(* Logix 5000 AddOnInstructionDefinition export SPEL_Init; software revision 30.01 *)

ADD_ON_INSTRUCTION SPEL_ExecCmd   (* revision 1.2 *)
// Executes a command in the robot controller.  Normally this is called by higher level AOIs.
VAR_INPUT
   Start : BOOL; {required}
   MaxTime : DINT := 3000; {required}
END_VAR
VAR_OUTPUT
   InCycle : BOOL; {access Read Only, visible}
   Done : BOOL; {access Read Only, visible}
   Error : BOOL; {access Read Only, visible}
END_VAR
VAR_IN_OUT
   ExtInputs : AB:ETHERNET_MODULE_INT_128Bytes:I:0; {required}
        .DATA[0].0   // ExtCmdGet
        .DATA[0].1   // ExtRespSet
        .DATA[0].2   // ExtCmdResult
        .DATA[0].3   // ExtError
   ExtOutputs : AB:ETHERNET_MODULE_INT_128Bytes:O:0; {required}
        .DATA[0].0   // ExtCmdSet
        .DATA[0].1   // ExtRespGet
        .DATA[0].2   // ExtCmdReset
END_VAR
VAR_INPUT
   Cmd : INT; {required}
   CmdParam1 : INT; {required}
   CmdParam2 : INT; {required}
   CmdParam3 : INT; {required}
   CmdParam4 : INT; {required}
   CmdParam5 : INT; {required}
   CmdParam6 : INT; {required}
   CmdParam7 : INT; {required}
END_VAR
VAR_OUTPUT
   CmdEcho : INT; {access Read Only, visible}
   Resp1 : INT; {access Read Only, visible}
   Resp2 : INT; {access Read Only, visible}
   Resp3 : INT; {access Read Only, visible}
   Resp4 : INT; {access Read Only, visible}
   Resp5 : INT; {access Read Only, visible}
   Resp6 : INT; {access Read Only, visible}
   Resp7 : INT; {access Read Only, visible}
   ErrCode1 : INT; {access Read Only, visible}
   ErrCode2 : INT; {access Read Only, visible}
END_VAR
VAR
   ExtReset : BOOL; {access None}
   ExtError : BOOL; {access None}
   ExtCmdSet : BOOL; {access None}   // Cmd Ready
   ExtCmdGet : BOOL; {access None}   // Cmd Received
   CmdXferDone : BOOL; {access None}
   ExtRespSet : BOOL; {access None}   // Resp Ready
   RespXferDone : BOOL; {access None}
   ExtCmdResult : BOOL; {access None}   // Normal or Error?
   TmrCmdDataRdy : TIMER := (PRE := 5); {access None}
   OneShotDoneOff : BOOL; {access None}
   OneShotStart : BOOL; {access None}
   StartInit : BOOL; {access None}
   OneShotStartError : BOOL; {access None}
   TmrCycle : TIMER := (PRE := 5000); {access None}
   OneshotTmrPreset : BOOL; {access None}
   TmrCmdSet : TIMER := (PRE := 20); {access None}
   OnShotCmdDataXfer : BOOL; {access None}
   OneShotRespDataXfer : BOOL; {access None}
   OneShotDataRdy : BOOL; {access None}
   OtherCmdInCycle : BOOL; {access None}
   s : BOOL; {access None}
   OneShotUnsetCmdIncycle : BOOL; {access None}
   OneShotSetCmdIncycle : BOOL; {access None}
   OneShotSetOtherCmdInCycleError : BOOL; {access None}
   OneShotSetBit : BOOL; {access None}
   MaxTimeError : BOOL; {access None}
END_VAR

ROUTINE Logic   (* ladder *)
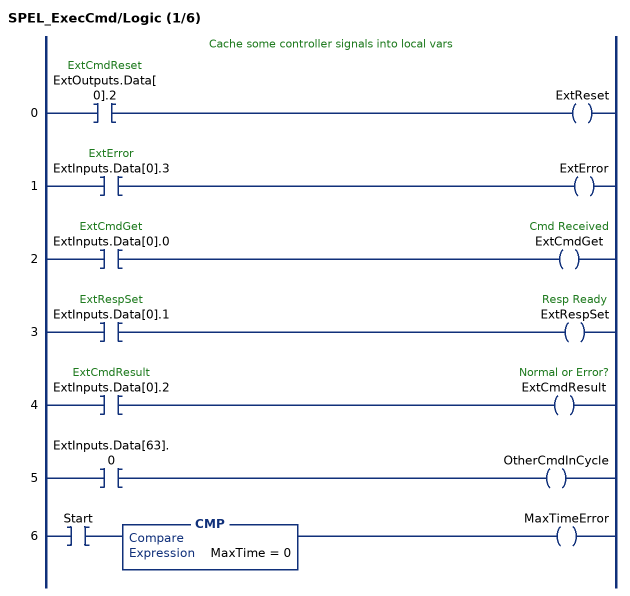
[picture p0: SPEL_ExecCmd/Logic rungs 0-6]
   // Cache some controller signals into local vars
   0: XIC(ExtOutputs.Data[0].2)OTE(ExtReset);
   1: XIC(ExtInputs.Data[0].3)OTE(ExtError);
   2: XIC(ExtInputs.Data[0].0)OTE(ExtCmdGet);
   3: XIC(ExtInputs.Data[0].1)OTE(ExtRespSet);
   4: XIC(ExtInputs.Data[0].2)OTE(ExtCmdResult);
   5: XIC(ExtInputs.Data[63].0)OTE(OtherCmdInCycle);
   6: XIC(Start)CMP(MaxTime = 0)OTE(MaxTimeError);
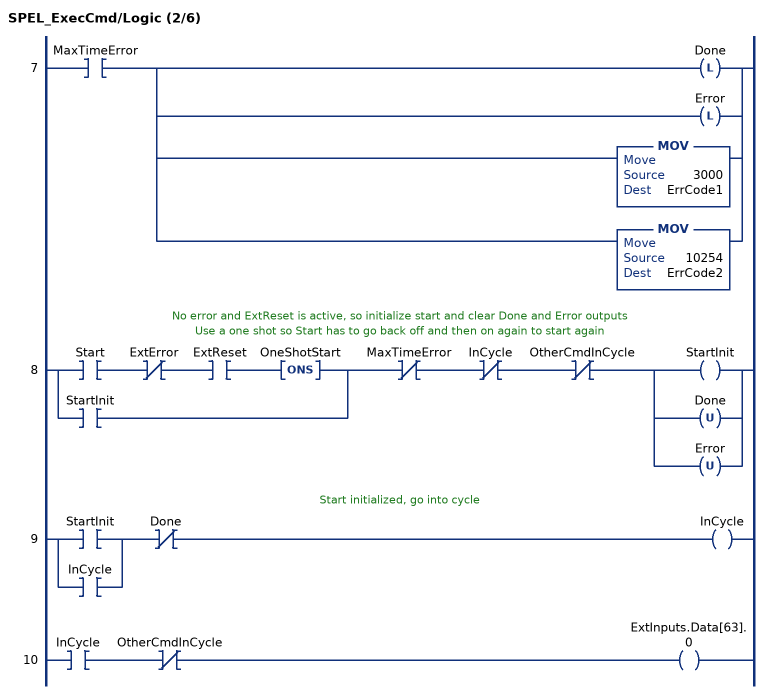
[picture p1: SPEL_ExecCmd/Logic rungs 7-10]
   7: XIC(MaxTimeError)[OTL(Done) ,OTL(Error) ,MOV(3000,ErrCode1) ,MOV(10254,ErrCode2) ];
   // No error and ExtReset is active, so initialize start and clear Done and Error outputs
   // Use a one shot so Start has to go back off and then on again to start again
   8: [XIC(Start) XIO(ExtError) XIC(ExtReset) ONS(OneShotStart) ,XIC(StartInit) ]XIO(MaxTimeError)XIO(InCycle)XIO(OtherCmdInCycle)[OTE(StartInit) ,OTU(Done) ,OTU(Error) ];
   // Start initialized, go into cycle
   9: [XIC(StartInit) ,XIC(InCycle) ]XIO(Done)OTE(InCycle);
   10: XIC(InCycle)XIO(OtherCmdInCycle)OTE(ExtInputs.Data[63].0);
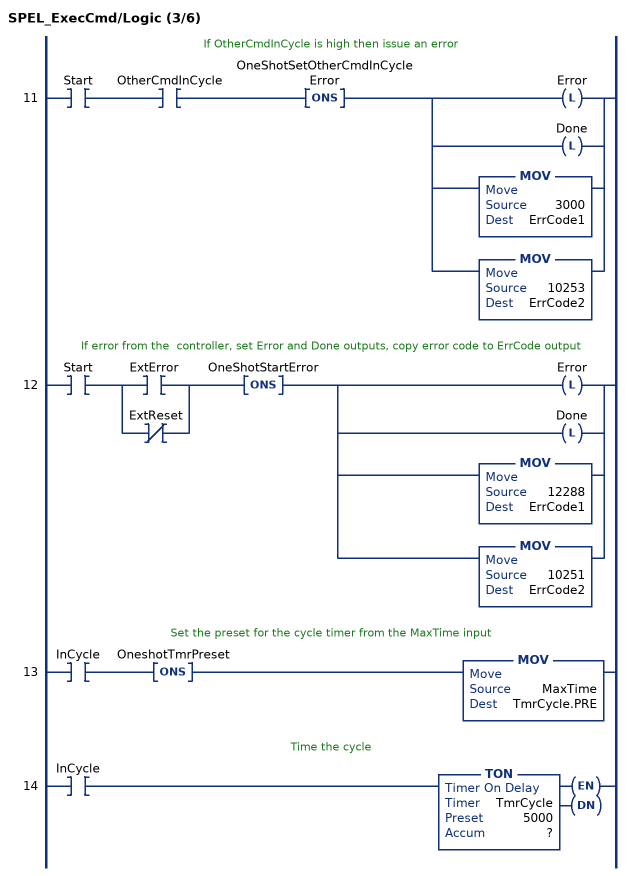
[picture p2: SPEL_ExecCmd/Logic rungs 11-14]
   // If OtherCmdInCycle is high then issue an error
   11: XIC(Start)XIC(OtherCmdInCycle)ONS(OneShotSetOtherCmdInCycleError)[OTL(Error) ,OTL(Done) ,MOV(3000,ErrCode1) ,MOV(10253,ErrCode2) ];
   // If error from the  controller, set Error and Done outputs, copy error code to ErrCode output
   12: XIC(Start)[XIC(ExtError) ,XIO(ExtReset) ]ONS(OneShotStartError)[OTL(Error) ,OTL(Done) ,MOV(12288,ErrCode1) ,MOV(10251,ErrCode2) ];
   // Set the preset for the cycle timer from the MaxTime input
   13: XIC(InCycle)ONS(OneshotTmrPreset)MOV(MaxTime,TmrCycle.PRE);
   // Time the cycle
   14: XIC(InCycle)TON(TmrCycle,?,?);
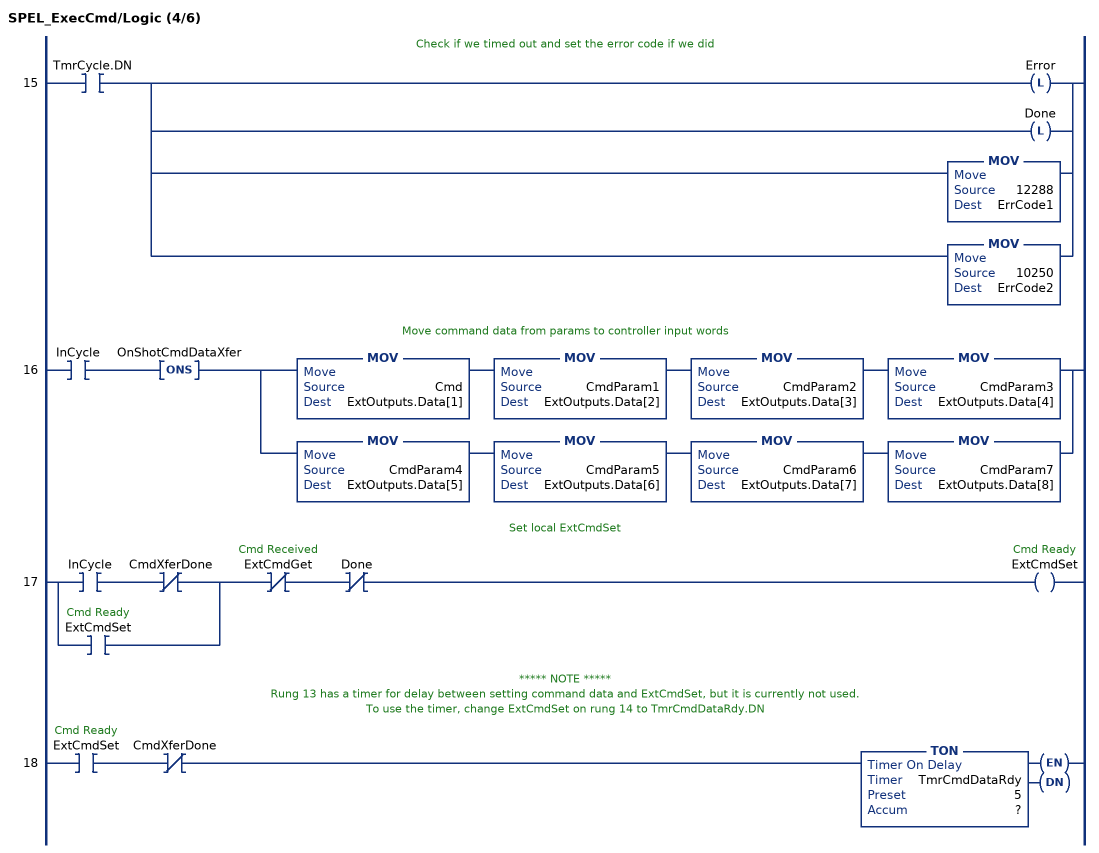
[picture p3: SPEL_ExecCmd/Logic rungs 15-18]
   // Check if we timed out and set the error code if we did
   15: XIC(TmrCycle.DN)[OTL(Error) ,OTL(Done) ,MOV(12288,ErrCode1) ,MOV(10250,ErrCode2) ];
   // Move command data from params to controller input words
   16: XIC(InCycle)ONS(OnShotCmdDataXfer)[MOV(Cmd,ExtOutputs.Data[1]) MOV(CmdParam1,ExtOutputs.Data[2]) MOV(CmdParam2,ExtOutputs.Data[3]) MOV(CmdParam3,ExtOutputs.Data[4]) ,MOV(CmdParam4,ExtOutputs.Data[5]) MOV(CmdParam5,ExtOutputs.Data[6]) MOV(CmdParam6,ExtOutputs.Data[7]) MOV(CmdParam7,ExtOutputs.Data[8]) ];
   // Set local ExtCmdSet
   17: [XIC(InCycle) XIO(CmdXferDone) ,XIC(ExtCmdSet) ]XIO(ExtCmdGet)XIO(Done)OTE(ExtCmdSet);
   // ***** NOTE *****
   // Rung 13 has a timer for delay between setting command data and ExtCmdSet, but it is currently not used.
   // To use the timer, change ExtCmdSet on rung 14 to TmrCmdDataRdy.DN
   18: XIC(ExtCmdSet)XIO(CmdXferDone)TON(TmrCmdDataRdy,?,?);
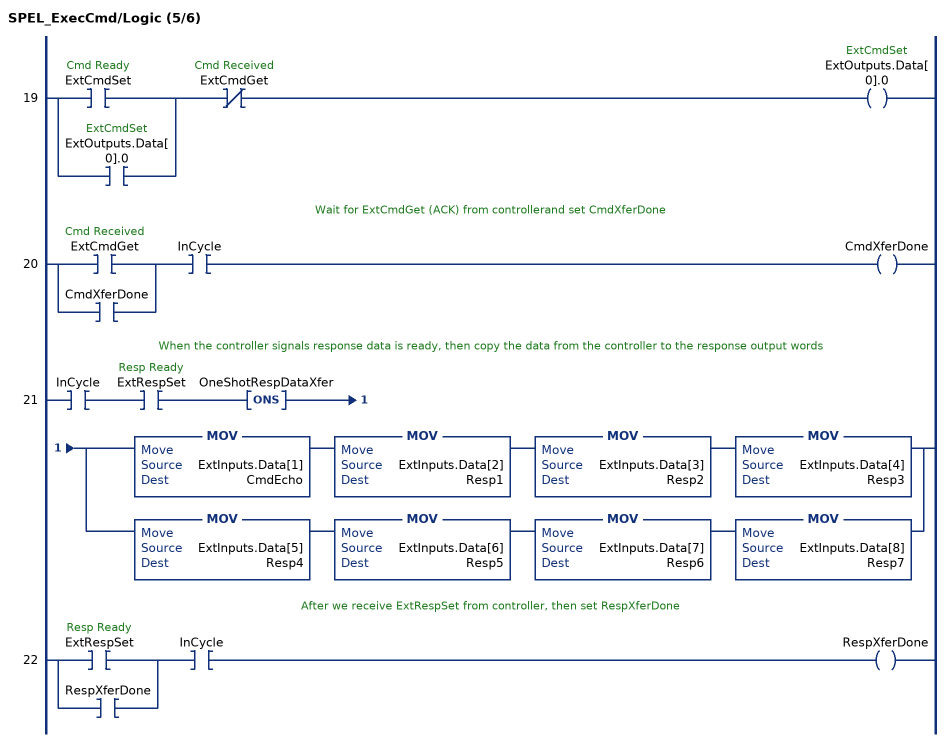
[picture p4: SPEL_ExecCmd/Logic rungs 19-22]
   19: [XIC(ExtCmdSet) ,XIC(ExtOutputs.Data[0].0) ]XIO(ExtCmdGet)OTE(ExtOutputs.Data[0].0);
   // Wait for ExtCmdGet (ACK) from controllerand set CmdXferDone
   20: [XIC(ExtCmdGet) ,XIC(CmdXferDone) ]XIC(InCycle)OTE(CmdXferDone);
   // When the controller signals response data is ready, then copy the data from the controller to the response output words
   21: XIC(InCycle)XIC(ExtRespSet)ONS(OneShotRespDataXfer)[MOV(ExtInputs.Data[1],CmdEcho) MOV(ExtInputs.Data[2],Resp1) MOV(ExtInputs.Data[3],Resp2) MOV(ExtInputs.Data[4],Resp3) ,MOV(ExtInputs.Data[5],Resp4) MOV(ExtInputs.Data[6],Resp5) MOV(ExtInputs.Data[7],Resp6) MOV(ExtInputs.Data[8],Resp7) ];
   // After we receive ExtRespSet from controller, then set RespXferDone
   22: [XIC(ExtRespSet) ,XIC(RespXferDone) ]XIC(InCycle)OTE(RespXferDone);
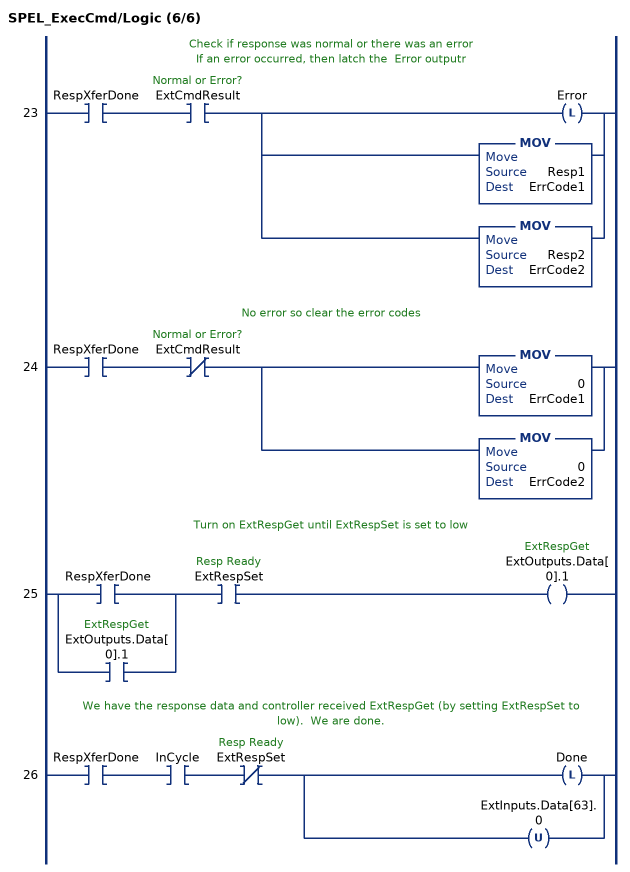
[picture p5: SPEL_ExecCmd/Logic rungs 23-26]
   // Check if response was normal or there was an error
   // If an error occurred, then latch the  Error outputr
   23: XIC(RespXferDone)XIC(ExtCmdResult)[OTL(Error) ,MOV(Resp1,ErrCode1) ,MOV(Resp2,ErrCode2) ];
   // No error so clear the error codes
   24: XIC(RespXferDone)XIO(ExtCmdResult)[MOV(0,ErrCode1) ,MOV(0,ErrCode2) ];
   // Turn on ExtRespGet until ExtRespSet is set to low
   25: [XIC(RespXferDone) ,XIC(ExtOutputs.Data[0].1) ]XIC(ExtRespSet)OTE(ExtOutputs.Data[0].1);
   // We have the response data and controller received ExtRespGet (by setting ExtRespSet to low).  We are done.
   26: XIC(RespXferDone)XIC(InCycle)XIO(ExtRespSet)[OTL(Done) ,OTU(ExtInputs.Data[63].0) ];
END_ROUTINE
END_ADD_ON_INSTRUCTION

ADD_ON_INSTRUCTION SPEL_ResetError   (* revision 1.0 *)
// Resets AOI library error state. This AOI must be executed to clear an error.
VAR_OUTPUT
   InCycle : BOOL; {access Read Only, visible}
   Done : BOOL; {visible}
   Error : BOOL; {access Read Only, visible}
END_VAR
VAR_INPUT
   Start : BOOL; {required}
END_VAR
VAR_IN_OUT
   ExtInputs : AB:ETHERNET_MODULE_INT_128Bytes:I:0; {required}
   ExtOutputs : AB:ETHERNET_MODULE_INT_128Bytes:O:0; {required}
END_VAR
VAR_OUTPUT
   ErrCode1 : INT; {access Read Only, visible}
   ErrCode2 : INT; {access Read Only, visible}
END_VAR
VAR
   TmrReset : TIMER := (PRE := 50); {access None}
   OneShotStart : BOOL; {access None}
   OneShotStart1 : BOOL; {access None}
   StartInit : BOOL; {access None}
   TmrWaitRdy : TIMER := (PRE := 100); {access None}
END_VAR

ROUTINE Logic   (* ladder *)
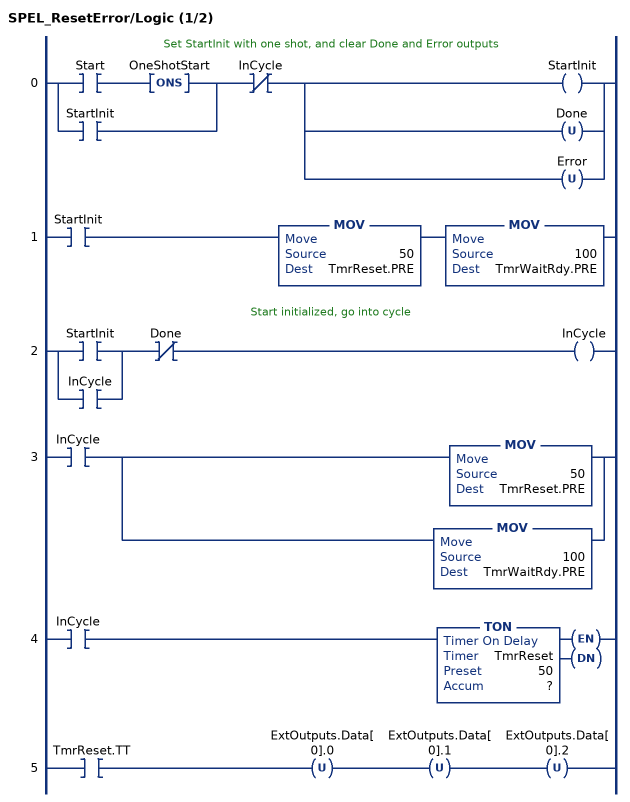
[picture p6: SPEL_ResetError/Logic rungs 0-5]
   // Set StartInit with one shot, and clear Done and Error outputs
   0: [XIC(Start) ONS(OneShotStart) ,XIC(StartInit) ]XIO(InCycle)[OTE(StartInit) ,[OTU(Done) ,OTU(Error) ] ];
   1: XIC(StartInit)MOV(50,TmrReset.PRE)MOV(100,TmrWaitRdy.PRE);
   // Start initialized, go into cycle
   2: [XIC(StartInit) ,XIC(InCycle) ]XIO(Done)OTE(InCycle);
   3: XIC(InCycle)[MOV(50,TmrReset.PRE) ,MOV(100,TmrWaitRdy.PRE) ];
   4: XIC(InCycle)TON(TmrReset,?,?);
   5: XIC(TmrReset.TT)OTU(ExtOutputs.Data[0].0)OTU(ExtOutputs.Data[0].1)OTU(ExtOutputs.Data[0].2);
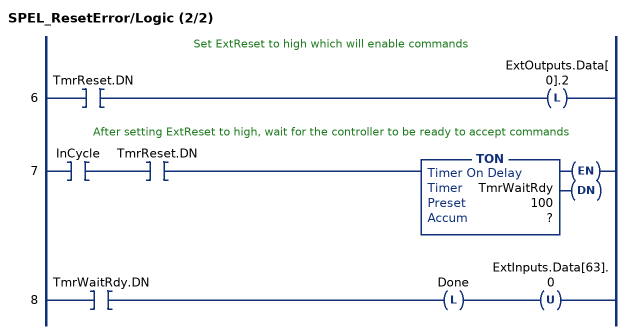
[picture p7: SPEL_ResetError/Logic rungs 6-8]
   // Set ExtReset to high which will enable commands
   6: XIC(TmrReset.DN)OTL(ExtOutputs.Data[0].2);
   // After setting ExtReset to high, wait for the controller to be ready to accept commands
   7: XIC(InCycle)XIC(TmrReset.DN)TON(TmrWaitRdy,?,?);
   8: XIC(TmrWaitRdy.DN)OTL(Done)OTU(ExtInputs.Data[63].0);
END_ROUTINE
END_ADD_ON_INSTRUCTION

ADD_ON_INSTRUCTION SPEL_Init   (* revision 1.2 *)
// Initialize the SPEL AOI library.
VAR_INPUT
   Start : BOOL; {required}
END_VAR
VAR_OUTPUT
   InCycle : BOOL; {access Read Only, visible}
   Done : BOOL; {access Read Only, visible}
   Error : BOOL; {access Read Only, visible}
END_VAR
VAR_IN_OUT
   ExtInputs : AB:ETHERNET_MODULE_INT_128Bytes:I:0; {required}
   ExtOutputs : AB:ETHERNET_MODULE_INT_128Bytes:O:0; {required}
END_VAR
VAR_OUTPUT
   ErrCode1 : INT; {access Read Only, visible}
   ErrCode2 : INT; {access Read Only, visible}
END_VAR
VAR
   ResetError : SPEL_ResetError; {access None}
        .INCYCLE   // ResetErrorInCycle
   ExecGetCCD : SPEL_ExecCmd := (MaxTime := 3000); {access None}
   RemoteIO_OK : BOOL; {access None}
   ExecGetPLC_ID : SPEL_ExecCmd := (MaxTime := 3000); {access None}
   AB_OK : BOOL; {access None}
   RemoteIO_Err : BOOL; {access None}
   AB_Err : BOOL; {access None}
   StartGetCCD : BOOL; {access None}
   StartGetCD_ONS : BOOL; {access None}
   Disable : BOOL; {access None}
   Disable2 : BOOL; {access None}
   TestStartCD : BOOL; {access None}
   TmrStartGetCD : TIMER := (PRE := 50); {access None}
   OneShotStartGetCCD : BOOL; {access None}
   StartGetPLC : BOOL; {access None}
   OneShotStartGetPLC : BOOL; {access None}
   ExecTimeout : DINT; {access None}
END_VAR

ROUTINE Logic   (* ladder *)
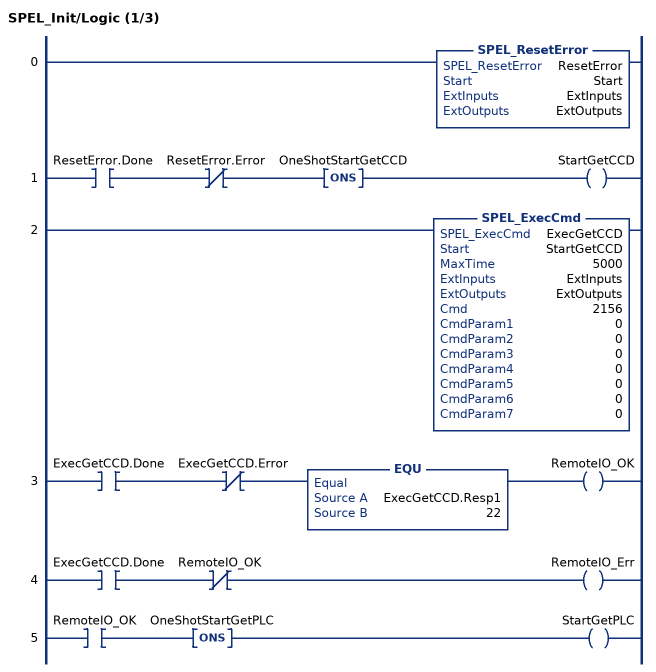
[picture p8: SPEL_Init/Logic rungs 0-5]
   0: SPEL_ResetError(ResetError,Start,ExtInputs,ExtOutputs);
   1: XIC(ResetError.Done)XIO(ResetError.Error)ONS(OneShotStartGetCCD)OTE(StartGetCCD);
   2: SPEL_ExecCmd(ExecGetCCD,StartGetCCD,5000,ExtInputs,ExtOutputs,2156,0,0,0,0,0,0,0);
   3: XIC(ExecGetCCD.Done)XIO(ExecGetCCD.Error)EQU(ExecGetCCD.Resp1,22)OTE(RemoteIO_OK);
   4: XIC(ExecGetCCD.Done)XIO(RemoteIO_OK)OTE(RemoteIO_Err);
   5: XIC(RemoteIO_OK)ONS(OneShotStartGetPLC)OTE(StartGetPLC);
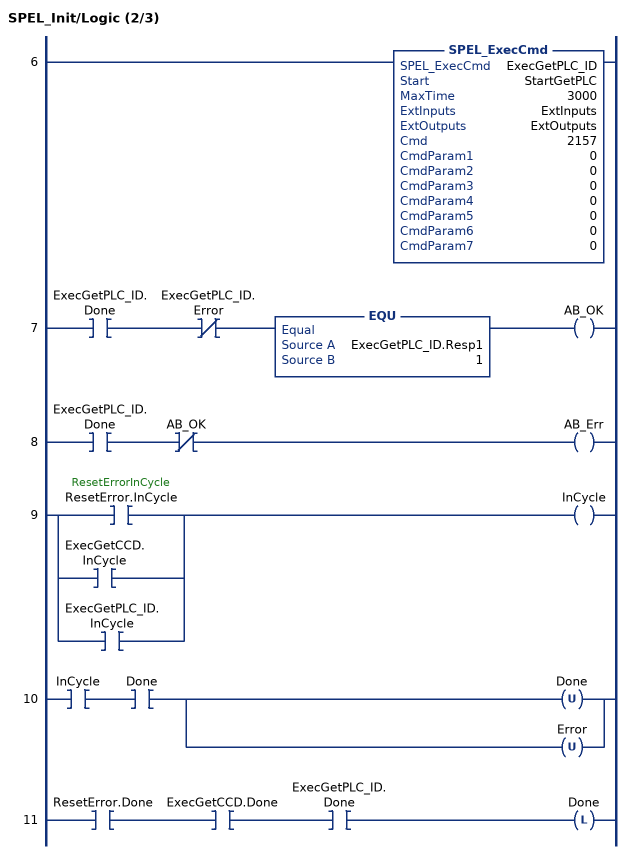
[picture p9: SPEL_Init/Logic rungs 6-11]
   6: SPEL_ExecCmd(ExecGetPLC_ID,StartGetPLC,3000,ExtInputs,ExtOutputs,2157,0,0,0,0,0,0,0);
   7: XIC(ExecGetPLC_ID.Done)XIO(ExecGetPLC_ID.Error)EQU(ExecGetPLC_ID.Resp1,1)OTE(AB_OK);
   8: XIC(ExecGetPLC_ID.Done)XIO(AB_OK)OTE(AB_Err);
   9: [XIC(ResetError.InCycle) ,XIC(ExecGetCCD.InCycle) ,XIC(ExecGetPLC_ID.InCycle) ]OTE(InCycle);
   10: XIC(InCycle)XIC(Done)[OTU(Done) ,OTU(Error) ];
   11: XIC(ResetError.Done)XIC(ExecGetCCD.Done)XIC(ExecGetPLC_ID.Done)OTL(Done);
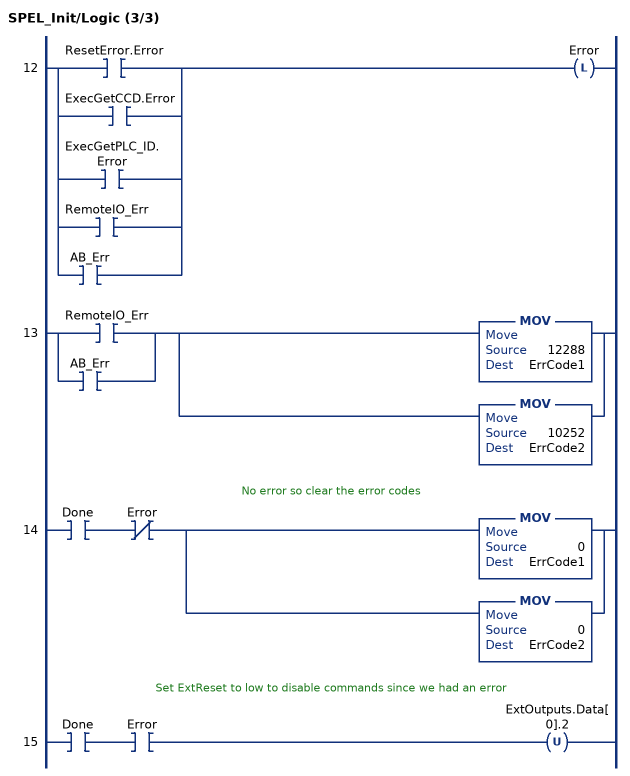
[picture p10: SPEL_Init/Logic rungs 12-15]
   12: [XIC(ResetError.Error) ,XIC(ExecGetCCD.Error) ,XIC(ExecGetPLC_ID.Error) ,XIC(RemoteIO_Err) ,XIC(AB_Err) ]OTL(Error);
   13: [XIC(RemoteIO_Err) ,XIC(AB_Err) ][MOV(12288,ErrCode1) ,MOV(10252,ErrCode2) ];
   // No error so clear the error codes
   14: XIC(Done)XIO(Error)[MOV(0,ErrCode1) ,MOV(0,ErrCode2) ];
   // Set ExtReset to low to disable commands since we had an error
   15: XIC(Done)XIC(Error)OTU(ExtOutputs.Data[0].2);
END_ROUTINE
END_ADD_ON_INSTRUCTION
